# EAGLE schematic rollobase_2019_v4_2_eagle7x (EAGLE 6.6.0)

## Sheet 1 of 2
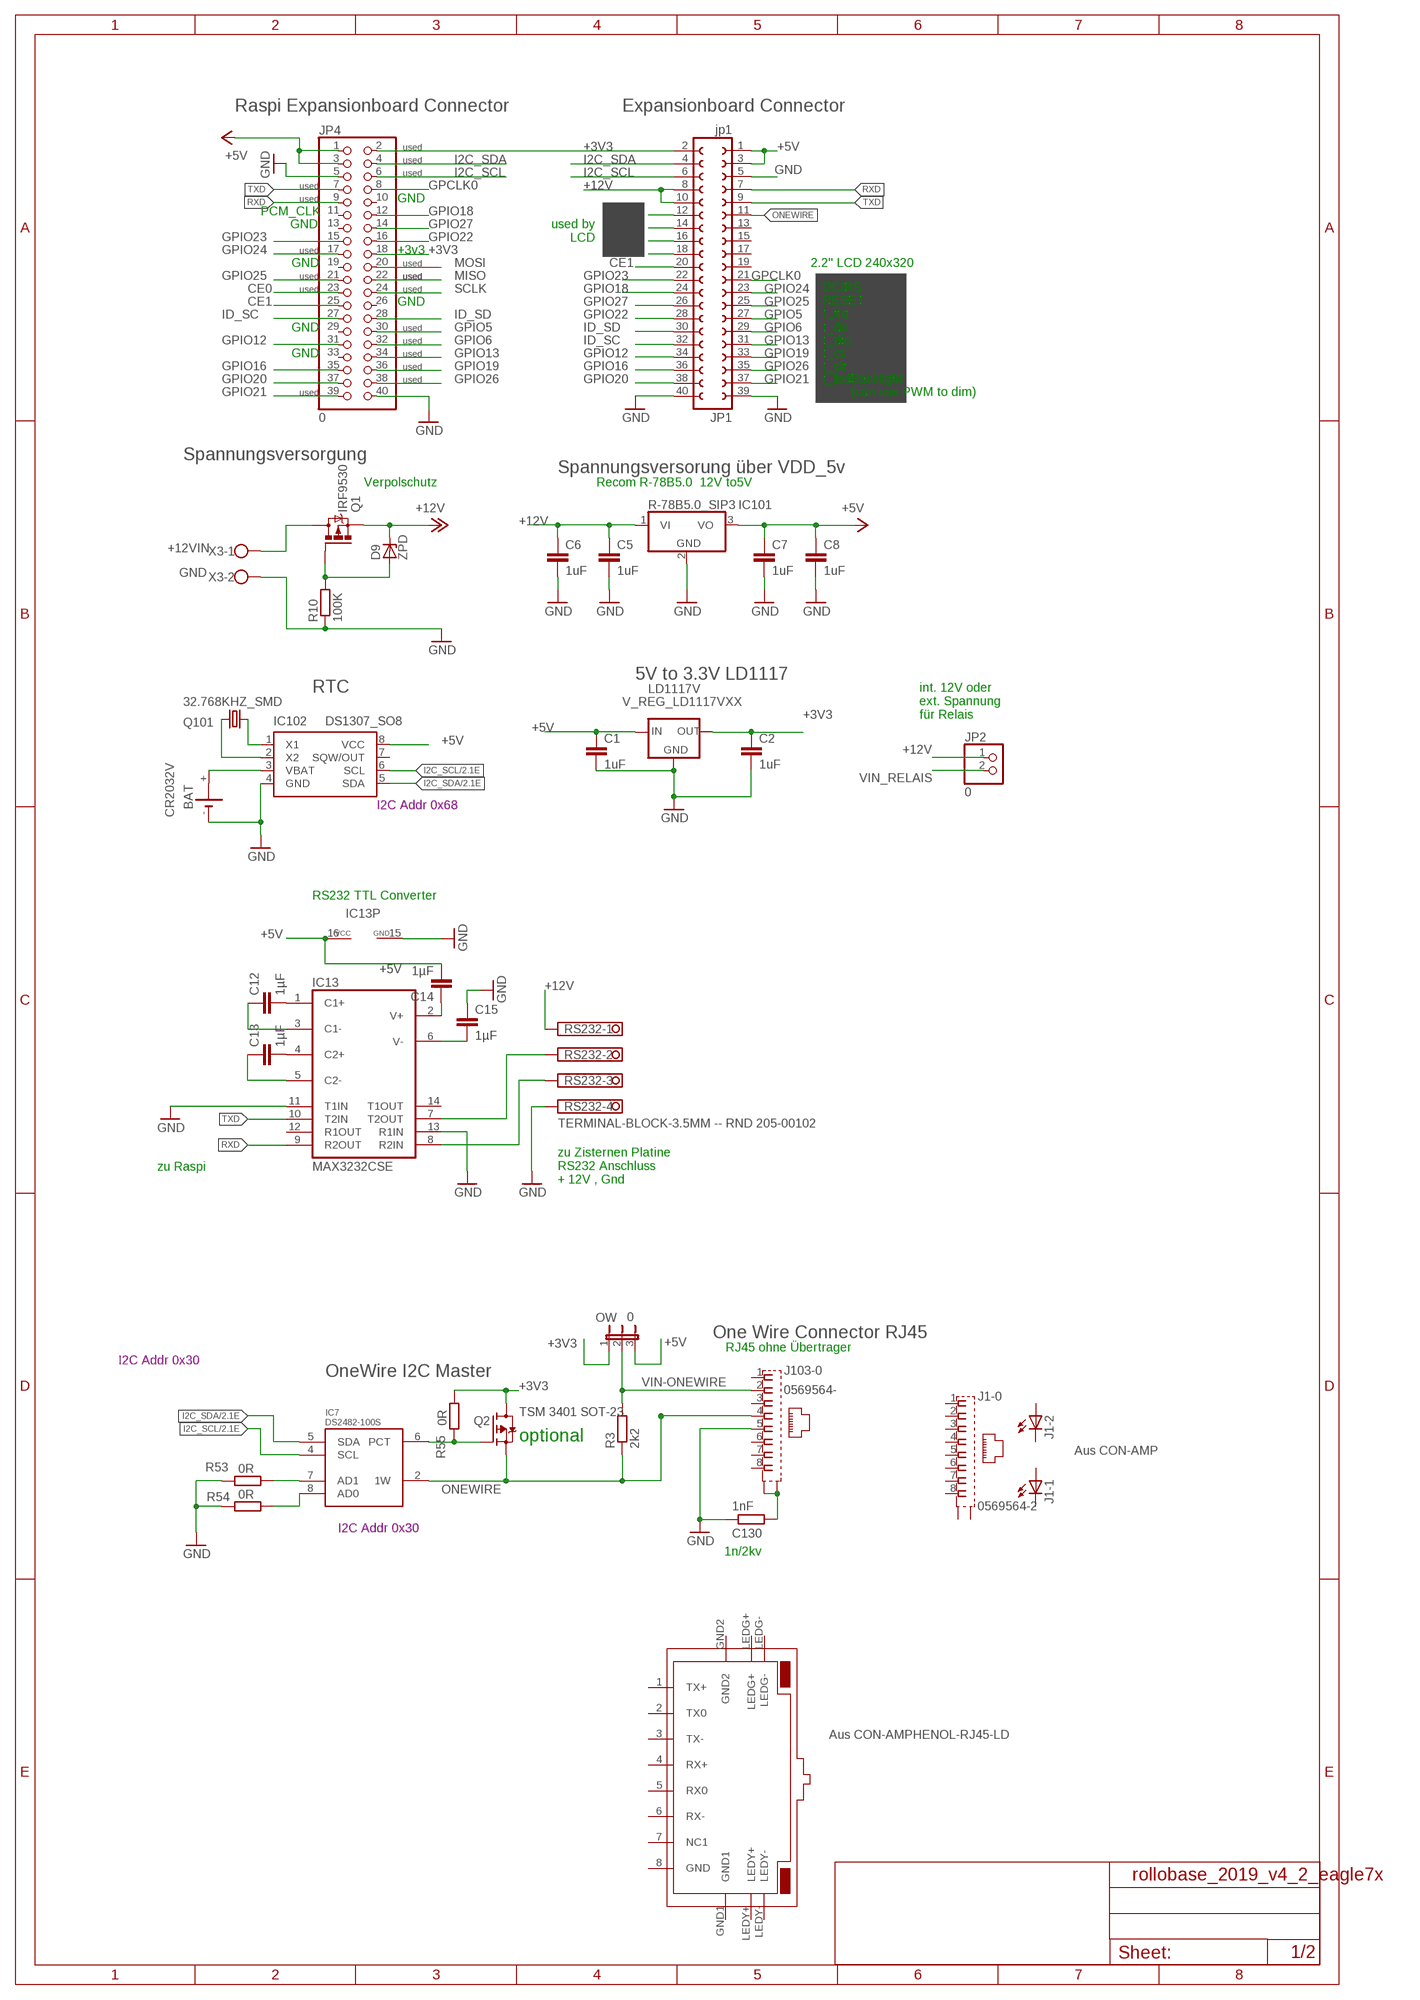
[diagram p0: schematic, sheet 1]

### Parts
BAT  CR2032V  [CR2032V]
C1  1uF  C-EUC1206  [C1206]
C2  1uF  C-EUC1206  [C1206]
C5  1uF  C-EUC1206  [C1206]
C6  1uF  C-EUC1206  [C1206]
C7  1uF  C-EUC1206  [C1206]
C8  1uF  C-EUC1206  [C1206]
C12  1µF  C-EUC1206  [C1206]
C13  1µF  C-EUC1206  [C1206]
C14  1µF  C-EUC1206  [C1206]
C15  1µF  C-EUC1206  [C1206]
C130  1nF  R-EU_R0805  [R0805]
D9  ZPD  [DO35Z10]
IC7  DS2482-100S  [SO08]
IC13  MAX3232CSE  [SO16]
IC101  R-78B5.0_SIP3  [SIP3]
IC102  DS1307_SO8  [SO08]
J1  0569564-2  [0569564]
J103  0569564-  [0569564]
JP1  jp1  FE20-2  [FE20-2]
JP2  0  PINHD-1X2  [1X02]
JP4  0  PINHD-2X20  [2X20]
LD1117V  V_REG_LD1117VXX  [78XXL]
OW  0  JP2E  [JP2]
Q1  IRF9530  [TO220BV]
Q2  TSM 3401 SOT-23  MOSFET-P-SOT23  [SOT23]
Q101  32.768KHZ_SMD  [QSMD]
R3  2k2  R-EU_M1206  [M1206]
R10  100K  R-EU_R1206  [R1206]
R53  0R  R-EU_R1206  [R1206]
R54  0R  R-EU_R1206  [R1206]
R55  0R  R-EU_R1206  [R1206]
RS232  TERMINAL-BLOCK-3.5MM -- RND 205-00102  TERMINAL-BLOCK-3.5MM-4-PIN-ROUND-PAD  [TERMINAL-BLOCK-4-PIN-3.5MM-ROUND-PAD]
U$3  RJ45-TRAFO-L  [RJ45-TRAFO-L]
X3  VERSORGUNG  W237-102  [W237-102]

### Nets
$N5555: C130.1 J103.S1(-0:S1) J103.S2(-0:S2)
+3V3: C2.1 JP1.2 JP4.2 JP4.18 LD1117V.GND(OUT) OW.1 Q2.3(D) R55.1 ; also sheet 2
+5V: C1.1 C7.1 C8.1 C14.2 IC13.16(VCC) IC101.3(VO) IC102.8(VCC) JP1.1 JP1.3 JP4.1 JP4.3 LD1117V.OUT(IN) OW.3
+12V: C5.1 C6.1 D9.C IC101.1(VI) JP1.8 JP1.10 JP2.1 Q1.S RS232.1
+12VIN: Q1.D X3.1
CE0: JP1.18 JP4.23
CE1: JP1.20 JP4.25
GND: BAT.- C1.2 C2.2 C5.2 C6.2 C7.2 C8.2 C15.1 C130.2 IC13.11(T1IN) IC13.13(R1IN) IC13.15(GND) IC101.2(GND) IC102.4(GND) J103.5 JP1.5 JP1.39 JP1.40 JP4.5 JP4.40 LD1117V.IN(GND) R10.1 R53.2 R54.2 RS232.4 X3.2 ; also sheet 2
GPCLK0: JP1.21 JP4.8
GPIO5: JP1.27 JP4.30
GPIO6: JP1.29 JP4.32
GPIO12: JP1.34 JP4.31
GPIO13: JP1.31 JP4.34
GPIO16: JP1.36 JP4.35
GPIO18: JP1.24 JP4.12
GPIO19: JP1.33 JP4.36
GPIO20: JP1.38 JP4.37
GPIO21: JP1.37 JP4.39
GPIO22: JP1.28 JP4.16
GPIO23: JP1.22 JP4.15
GPIO24: JP1.23 JP4.17
GPIO25: JP1.25 JP4.21
GPIO26: JP1.35 JP4.38
GPIO27: JP1.26 JP4.14
I2C_SCL: IC7.4(SCL) IC102.6(SCL) JP1.6 JP4.6 ; also sheet 2
I2C_SDA: IC7.5(SDA) IC102.5(SDA) JP1.4 JP4.4 ; also sheet 2
ID_SC: JP1.32 JP4.27
ID_SD: JP1.30 JP4.28
MISO: JP1.14 JP4.22
MOSI: JP1.12 JP4.20
N$1: IC7.7(AD1) R53.1
N$2: IC7.8(AD0) R54.1
N$12: BAT.+ IC102.3(VBAT)
N$27: IC102.2(X2) Q101.1
N$29: IC102.1(X1) Q101.2
N$35: C12.2 IC13.1(C1+)
N$36: C13.2 IC13.4(C2+)
N$39: C14.1 IC13.2(V+)
N$43: C15.2 IC13.6(V-)
N$44: D9.A Q1.G R10.2
N$52: C12.1 IC13.3(C1-)
N$54: C13.1 IC13.5(C2-)
ONEWIRE: IC7.2(1W) J103.4 JP1.11 Q2.2(S) R3.1
PCTLZ: IC7.6(PCT) Q2.1(G) R55.2
RX: IC13.8(R2IN) RS232.3
RXD: IC13.9(R2OUT) JP1.7 JP4.9
SCLK: JP1.16 JP4.24
TX: IC13.7(T2OUT) RS232.2
TXD: IC13.10(T2IN) JP1.9 JP4.7
VIN-ONEWIRE: J103.2 OW.2 R3.2
VIN_RELAIS: JP2.2 ; also sheet 2
Unconnected: BAT.+@1(+) IC13.12(R1OUT) IC13.14(T1OUT) IC102.7(SQW/OUT) J1.1 J1.2 J1.3 J1.4 J1.5 J1.6 J1.7 J1.8 J1.A1(-1:A) J1.A2(-2:A) J1.C1(-1:C) J1.C2(-2:C) J1.S1(-0:S1) J1.S2(-0:S2) J103.1 J103.3 J103.6 J103.7 J103.8 J103.A1(-1:A) J103.A2(-2:A) J103.C1(-1:C) J103.C2(-2:C) JP1.13 JP1.15 JP1.17 JP1.19 JP4.10 JP4.11 JP4.13 JP4.19 JP4.26 JP4.29 JP4.33 U$3.1(TX+) U$3.2(TX0) U$3.3(TX-) U$3.4(RX+) U$3.5(RX0) U$3.6(RX-) U$3.7(NC1) U$3.LEDG+ U$3.LEDG- U$3.LEDY+ U$3.LEDY-

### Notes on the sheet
- Raspi Expansionboard Connector | Expansionboard Connector
- used
- used
- used
- used
- used | GND
- PCM_CLK
- used by
       LCD
- GND
- used | +3v3
- GND | used | 2.2'' LCD 240x320
- used | used | used
- used | used | DC/RS
- GND | RESET
- t_irq
- GND | used | t_do
- used | t_dio
- GND | used | t_cs
- used | t_clr
- used | t_led
- used
- Backlight
  (can use PWM to dim)
- Spannungsversorgung
- Spannungsversorung über VDD_5v
- Verpolschutz | Recom R-78B5.0 | 12V to5V
- 5V to 3.3V LD1117
- RTC
- int. 12V oder
  ext. Spannung 
  für Relais
- I2C Addr 0x68
- RS232 TTL Converter
- zu Raspi
- zu Zisternen Platine
  RS232 Anschluss
  + 12V , Gnd
- One Wire Connector RJ45
- RJ45 ohne Übertrager
- I2C Addr 0x30
- OneWire I2C Master
- optional
- Aus CON-AMP
- I2C Addr 0x30
- 1n/2kv
- Aus CON-AMPHENOL-RJ45-LD

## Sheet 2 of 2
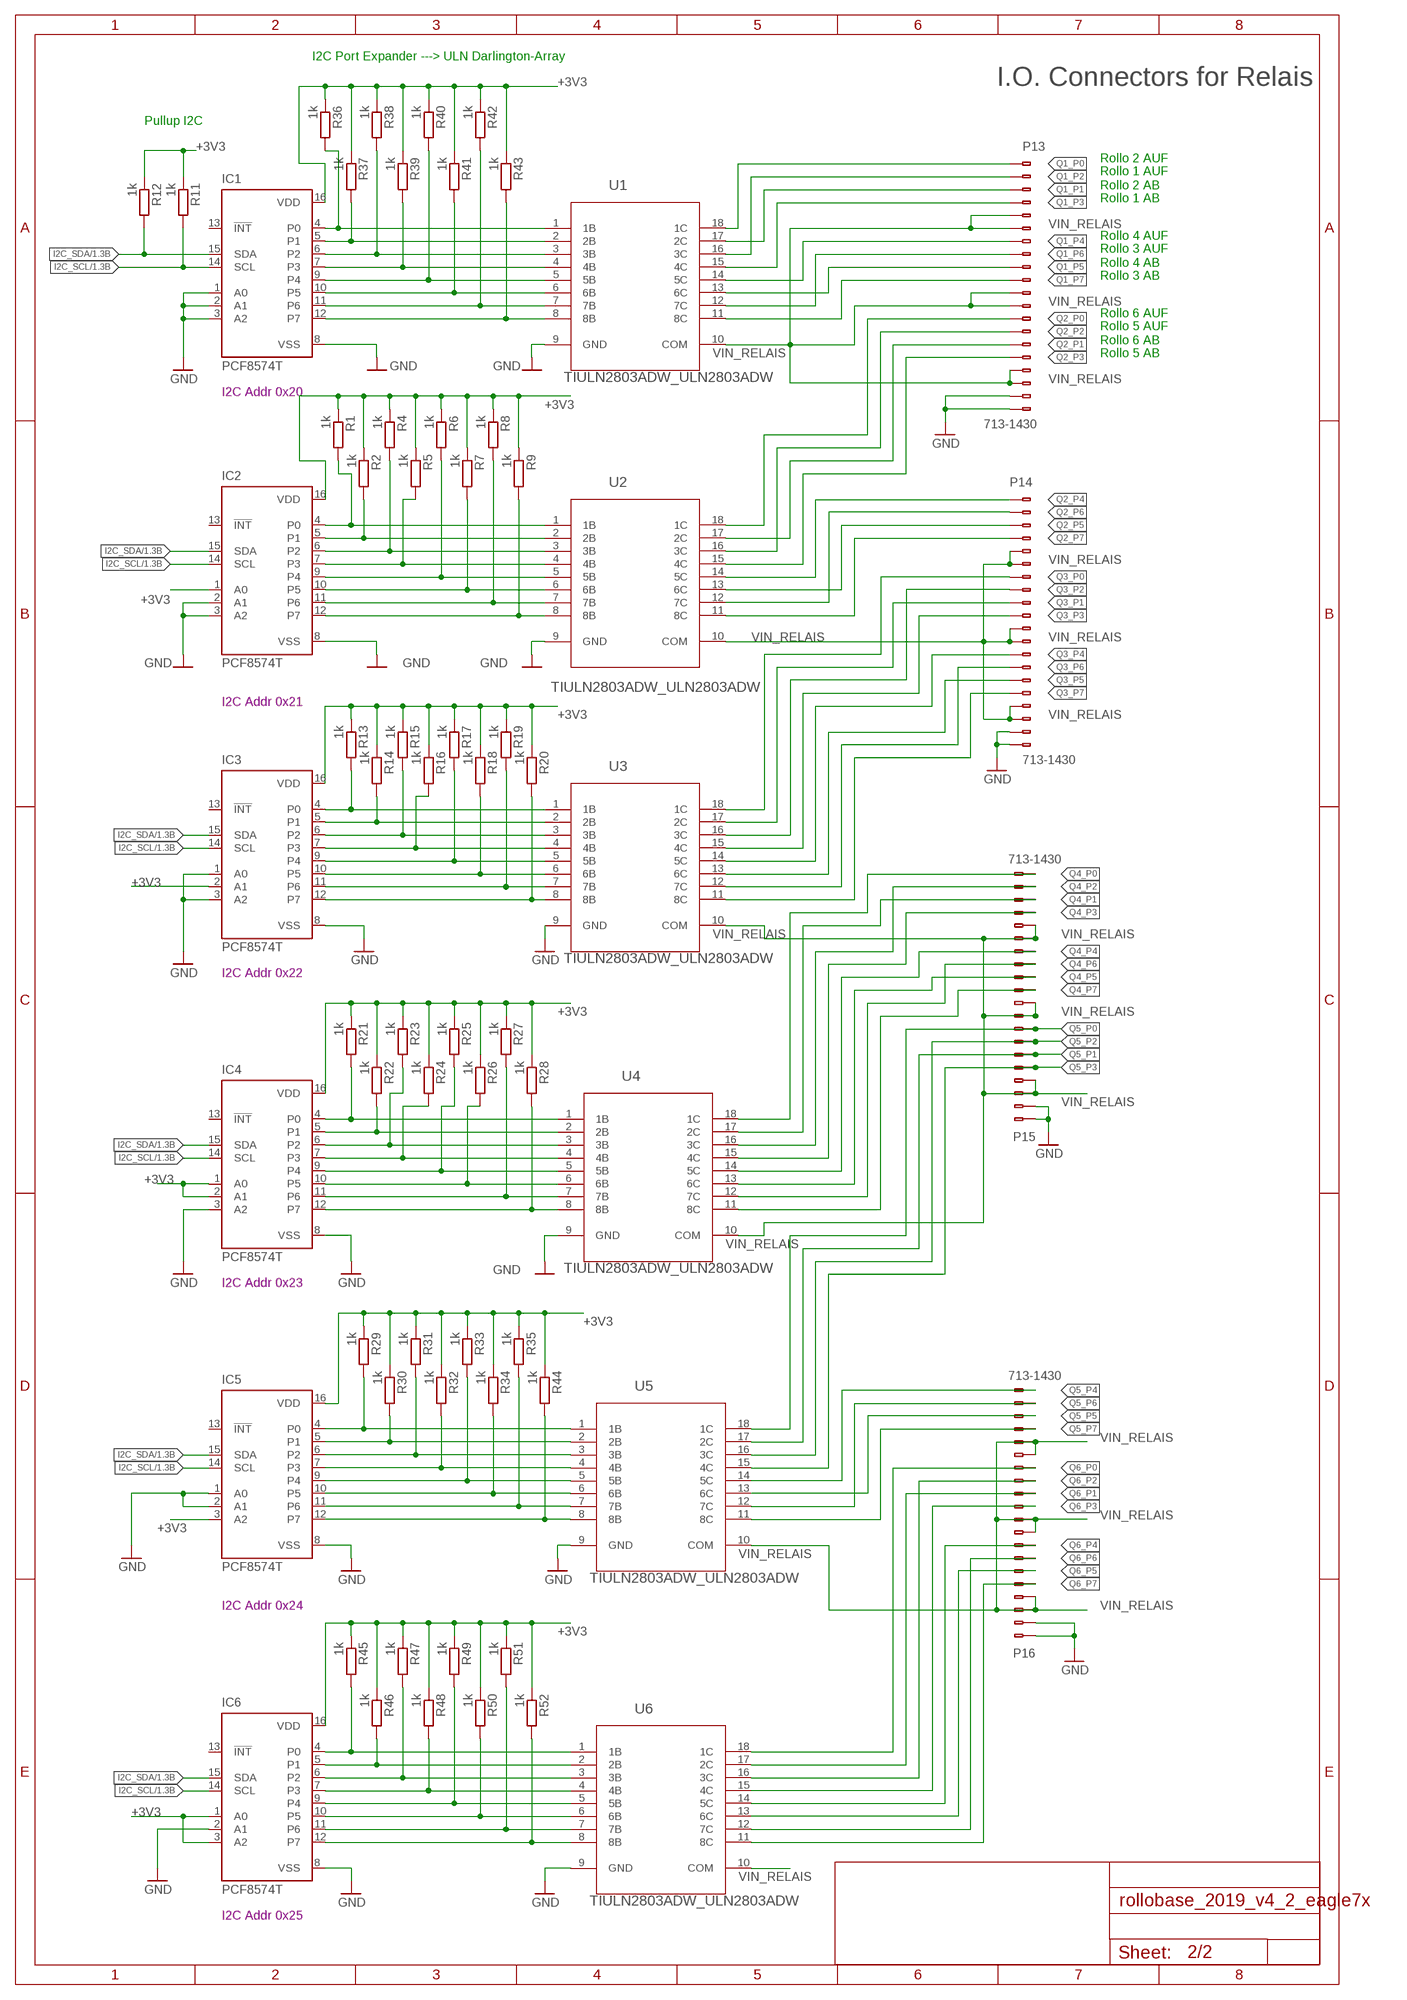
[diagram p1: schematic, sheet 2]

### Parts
IC1  PCF8574T  [SO16W]
IC2  PCF8574T  [SO16W]
IC3  PCF8574T  [SO16W]
IC4  PCF8574T  [SO16W]
IC5  PCF8574T  [SO16W]
IC6  PCF8574T  [SO16W]
P13  713-1430  [713-1425]
P14  713-1430  [713-1425]
P15  713-1430  [713-1425]
P16  713-1430  [713-1425]
R1  1k  R-EU_R0805  [R0805]
R2  1k  R-EU_R0805  [R0805]
R4  1k  R-EU_R0805  [R0805]
R5  1k  R-EU_R0805  [R0805]
R6  1k  R-EU_R0805  [R0805]
R7  1k  R-EU_R0805  [R0805]
R8  1k  R-EU_R0805  [R0805]
R9  1k  R-EU_R0805  [R0805]
R11  1k  R-EU_R1206  [R1206]
R12  1k  R-EU_R1206  [R1206]
R13  1k  R-EU_R0805  [R0805]
R14  1k  R-EU_R0805  [R0805]
R15  1k  R-EU_R0805  [R0805]
R16  1k  R-EU_R0805  [R0805]
R17  1k  R-EU_R0805  [R0805]
R18  1k  R-EU_R0805  [R0805]
R19  1k  R-EU_R0805  [R0805]
R20  1k  R-EU_R0805  [R0805]
R21  1k  R-EU_R0805  [R0805]
R22  1k  R-EU_R0805  [R0805]
R23  1k  R-EU_R0805  [R0805]
R24  1k  R-EU_R0805  [R0805]
R25  1k  R-EU_R0805  [R0805]
R26  1k  R-EU_R0805  [R0805]
R27  1k  R-EU_R0805  [R0805]
R28  1k  R-EU_R0805  [R0805]
R29  1k  R-EU_R0805  [R0805]
R30  1k  R-EU_R0805  [R0805]
R31  1k  R-EU_R0805  [R0805]
R32  1k  R-EU_R0805  [R0805]
R33  1k  R-EU_R0805  [R0805]
R34  1k  R-EU_R0805  [R0805]
R35  1k  R-EU_R0805  [R0805]
R36  1k  R-EU_R0805  [R0805]
R37  1k  R-EU_R0805  [R0805]
R38  1k  R-EU_R0805  [R0805]
R39  1k  R-EU_R0805  [R0805]
R40  1k  R-EU_R0805  [R0805]
R41  1k  R-EU_R0805  [R0805]
R42  1k  R-EU_R0805  [R0805]
R43  1k  R-EU_R0805  [R0805]
R44  1k  R-EU_R0805  [R0805]
R45  1k  R-EU_R0805  [R0805]
R46  1k  R-EU_R0805  [R0805]
R47  1k  R-EU_R0805  [R0805]
R48  1k  R-EU_R0805  [R0805]
R49  1k  R-EU_R0805  [R0805]
R50  1k  R-EU_R0805  [R0805]
R51  1k  R-EU_R0805  [R0805]
R52  1k  R-EU_R0805  [R0805]
U1  TIULN2803ADW_ULN2803ADW  [TIULN2803ADW_SOIC127P1030X265-18N]
U2  TIULN2803ADW_ULN2803ADW  [TIULN2803ADW_SOIC127P1030X265-18N]
U3  TIULN2803ADW_ULN2803ADW  [TIULN2803ADW_SOIC127P1030X265-18N]
U4  TIULN2803ADW_ULN2803ADW  [TIULN2803ADW_SOIC127P1030X265-18N]
U5  TIULN2803ADW_ULN2803ADW  [TIULN2803ADW_SOIC127P1030X265-18N]
U6  TIULN2803ADW_ULN2803ADW  [TIULN2803ADW_SOIC127P1030X265-18N]

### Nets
+3V3: IC1.16(VDD) IC2.1(A0) IC2.16(VDD) IC3.2(A1) IC3.16(VDD) IC4.1(A0) IC4.2(A1) IC4.16(VDD) IC5.3(A2) IC5.16(VDD) IC6.1(A0) IC6.3(A2) IC6.16(VDD) R1.1 R2.1 R4.1 R5.1 R6.1 R7.1 R8.1 R9.1 R11.1 R12.1 R13.1 R14.1 R15.1 R16.1 R17.1 R18.1 R19.1 R20.1 R21.1 R22.1 R23.1 R24.1 R25.1 R26.1 R27.1 R28.1 R29.1 R30.1 R31.1 R32.1 R33.1 R34.1 R35.1 R36.1 R37.1 R38.1 R39.1 R40.1 R41.1 R42.1 R43.1 R44.1 R45.1 R46.1 R47.1 R48.1 R49.1 R50.1 R51.1 R52.1 ; also sheet 1
GND: IC1.1(A0) IC1.2(A1) IC1.3(A2) IC1.8(VSS) IC2.2(A1) IC2.3(A2) IC2.8(VSS) IC3.1(A0) IC3.3(A2) IC3.8(VSS) IC4.3(A2) IC4.8(VSS) IC5.1(A0) IC5.2(A1) IC5.8(VSS) IC6.2(A1) IC6.8(VSS) P13.19(B-19) P13.20(B-20) P14.19(B-19) P14.20(B-20) P15.1(B-1) P15.2(B-2) P16.1(B-1) P16.2(B-2) U1.9(GND) U2.9(GND) U3.9(GND) U4.9(GND) U5.9(GND) U6.9(GND) ; also sheet 1
I2C_SCL: IC1.14(SCL) IC2.14(SCL) IC3.14(SCL) IC4.14(SCL) IC5.14(SCL) IC6.14(SCL) R11.2 ; also sheet 1
I2C_SDA: IC1.15(SDA) IC2.15(SDA) IC3.15(SDA) IC4.15(SDA) IC5.15(SDA) IC6.15(SDA) R12.2 ; also sheet 1
IC1_P1: IC1.5(P1) R37.2 U1.2(2B)
IC1_P2: IC2.5(P1) R2.2 U2.2(2B)
IC1_P3: IC2.4(P0) R1.2 U2.1(1B)
IC1_P4: IC2.6(P2) R4.2 U2.3(3B)
IC1_P5: IC2.7(P3) R5.2 U2.4(4B)
IC1_P6: IC2.9(P4) R6.2 U2.5(5B)
IC1_P7: IC2.10(P5) R7.2 U2.6(6B)
IC1_P8: IC2.11(P6) R8.2 U2.7(7B)
IC1_P9: IC1.4(P0) R36.2 U1.1(1B)
IC1_P10: IC1.6(P2) R38.2 U1.3(3B)
IC1_P11: IC1.7(P3) R39.2 U1.4(4B)
IC1_P12: IC1.9(P4) R40.2 U1.5(5B)
IC1_P13: IC1.10(P5) R41.2 U1.6(6B)
IC1_P14: IC1.11(P6) R42.2 U1.7(7B)
IC1_P15: IC1.12(P7) R43.2 U1.8(8B)
IC1_P16: IC2.12(P7) R9.2 U2.8(8B)
IC1_P17: IC3.5(P1) R14.2 U3.2(2B)
IC1_P18: IC3.4(P0) R13.2 U3.1(1B)
IC1_P19: IC3.6(P2) R15.2 U3.3(3B)
IC1_P20: IC3.7(P3) R16.2 U3.4(4B)
IC1_P21: IC3.9(P4) R17.2 U3.5(5B)
IC1_P22: IC3.10(P5) R18.2 U3.6(6B)
IC1_P23: IC3.11(P6) R19.2 U3.7(7B)
IC1_P24: IC3.12(P7) R20.2 U3.8(8B)
IC1_P25: IC4.5(P1) R22.2 U4.2(2B)
IC1_P26: IC4.4(P0) R21.2 U4.1(1B)
IC1_P27: IC4.6(P2) R23.2 U4.3(3B)
IC1_P28: IC4.7(P3) R24.2 U4.4(4B)
IC1_P29: IC4.9(P4) R25.2 U4.5(5B)
IC1_P30: IC4.10(P5) R26.2 U4.6(6B)
IC1_P31: IC4.11(P6) R27.2 U4.7(7B)
IC1_P32: IC4.12(P7) R28.2 U4.8(8B)
IC1_P33: IC5.5(P1) R30.2 U5.2(2B)
IC1_P34: IC5.4(P0) R29.2 U5.1(1B)
IC1_P35: IC5.6(P2) R31.2 U5.3(3B)
IC1_P36: IC5.7(P3) R32.2 U5.4(4B)
IC1_P37: IC5.9(P4) R33.2 U5.5(5B)
IC1_P38: IC5.10(P5) R34.2 U5.6(6B)
IC1_P39: IC5.11(P6) R35.2 U5.7(7B)
IC1_P40: IC5.12(P7) R44.2 U5.8(8B)
IC6_P0: IC6.4(P0) R45.2 U6.1(1B)
IC6_P1: IC6.5(P1) R46.2 U6.2(2B)
IC6_P2: IC6.6(P2) R47.2 U6.3(3B)
IC6_P3: IC6.7(P3) R48.2 U6.4(4B)
IC6_P4: IC6.9(P4) R49.2 U6.5(5B)
IC6_P5: IC6.10(P5) R50.2 U6.6(6B)
IC6_P6: IC6.11(P6) R51.2 U6.7(7B)
IC6_P7: IC6.12(P7) R52.2 U6.8(8B)
Q1_P0: P13.1(B-1) U1.18(1C)
Q1_P1: P13.3(B-3) U1.17(2C)
Q1_P2: P13.2(B-2) U1.16(3C)
Q1_P3: P13.4(B-4) U1.15(4C)
Q1_P4: P13.7(B-7) U1.14(5C)
Q1_P5: P13.9(B-9) U1.13(6C)
Q1_P6: P13.8(B-8) U1.12(7C)
Q1_P7: P13.10(B-10) U1.11(8C)
Q2_P0: P13.13(B-13) U2.18(1C)
Q2_P1: P13.15(B-15) U2.17(2C)
Q2_P2: P13.14(B-14) U2.16(3C)
Q2_P3: P13.16(B-16) U2.15(4C)
Q2_P4: P14.1(B-1) U2.14(5C)
Q2_P5: P14.3(B-3) U2.13(6C)
Q2_P6: P14.2(B-2) U2.12(7C)
Q2_P7: P14.4(B-4) U2.11(8C)
Q3_P0: P14.7(B-7) U3.18(1C)
Q3_P1: P14.9(B-9) U3.17(2C)
Q3_P2: P14.8(B-8) U3.16(3C)
Q3_P3: P14.10(B-10) U3.15(4C)
Q3_P4: P14.13(B-13) U3.14(5C)
Q3_P5: P14.15(B-15) U3.13(6C)
Q3_P6: P14.14(B-14) U3.12(7C)
Q3_P7: P14.16(B-16) U3.11(8C)
Q4_P0: P15.20(B-20) U4.18(1C)
Q4_P1: P15.18(B-18) U4.17(2C)
Q4_P2: P15.19(B-19) U4.16(3C)
Q4_P3: P15.17(B-17) U4.15(4C)
Q4_P4: P15.14(B-14) U4.14(5C)
Q4_P5: P15.12(B-12) U4.13(6C)
Q4_P6: P15.13(B-13) U4.12(7C)
Q4_P7: P15.11(B-11) U4.11(8C)
Q5_P0: P15.8(B-8) U5.18(1C)
Q5_P1: P15.6(B-6) U5.17(2C)
Q5_P2: P15.7(B-7) U5.16(3C)
Q5_P3: P15.5(B-5) U5.15(4C)
Q5_P4: P16.20(B-20) U5.14(5C)
Q5_P5: P16.18(B-18) U5.13(6C)
Q5_P6: P16.19(B-19) U5.12(7C)
Q5_P7: P16.17(B-17) U5.11(8C)
Q6_P0: P16.14(B-14) U6.18(1C)
Q6_P1: P16.12(B-12) U6.17(2C)
Q6_P2: P16.13(B-13) U6.16(3C)
Q6_P3: P16.11(B-11) U6.15(4C)
Q6_P4: P16.8(B-8) U6.14(5C)
Q6_P5: P16.6(B-6) U6.13(6C)
Q6_P6: P16.7(B-7) U6.12(7C)
Q6_P7: P16.5(B-5) U6.11(8C)
VIN_RELAIS: P13.5(B-5) P13.6(B-6) P13.11(B-11) P13.12(B-12) P13.17(B-17) P13.18(B-18) P14.5(B-5) P14.6(B-6) P14.11(B-11) P14.12(B-12) P14.17(B-17) P14.18(B-18) P15.3(B-3) P15.4(B-4) P15.9(B-9) P15.10(B-10) P15.15(B-15) P15.16(B-16) P16.3(B-3) P16.4(B-4) P16.9(B-9) P16.10(B-10) P16.15(B-15) P16.16(B-16) U1.10(COM) U2.10(COM) U3.10(COM) U4.10(COM) U5.10(COM) U6.10(COM) ; also sheet 1
Unconnected: IC1.13(!INT) IC2.13(!INT) IC3.13(!INT) IC4.13(!INT) IC5.13(!INT) IC6.13(!INT)

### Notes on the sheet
- I2C Port Expander ---> ULN Darlington-Array
- I.O. Connectors for Relais
- Pullup I2C
- Rollo 2 AUF
  
  Rollo 2 AB
- Rollo 1 AUF
  
  Rollo 1 AB
- Rollo 4 AUF
  
  Rollo 4 AB
- Rollo 3 AUF
  
  Rollo 3 AB
- Rollo 6 AUF
  
  Rollo 6 AB
- Rollo 5 AUF
  
  Rollo 5 AB
- I2C Addr 0x20
- I2C Addr 0x21
- I2C Addr 0x22
- I2C Addr 0x23
- I2C Addr 0x24
- I2C Addr 0x25

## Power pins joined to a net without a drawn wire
GND: IC7.3(GND) U$3.8(GND)
GND1: U$3.GND1
GND2: U$3.GND2
VDD: IC7.1(VDD)

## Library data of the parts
BAT = battery:CR2032V: LI BATTERY Varta
C1 C2 C5-C8 = resistor:C-EU: CAPACITOR, European symbol
C12-C15 = rcl:C-EU: CAPACITOR, European symbol
C130 R10-R12 R53-R55 = resistor:R-EU_: RESISTOR, European symbol
D9 = diode:ZPD: Z DIODE
IC1-IC6 = micro-philips:PCF8574: I2C-Bus Remote 8-bit I/O expander http://www.semiconductors.philips.com/acrobat_download/datasheets/PCF8574_4.pdf; MPN: PCF8574T/3,512; OC_FARNELL: 1201255; OC_NEWARK: 70R6870
IC7 = 1wire:DS2482-100: I2C to 1-Wire Host Adapter/Line Driver This device is a onewire host and I2C interface in one chip. It provides the complete DC/AC requirements for onewire communication, including overdrive speed mode, but, unlike the DS2480B chip, no 12V EPROM programming. Notes: For overdrive speed and 5V EEPROM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
IC13 = maxim:MAX3232*: True RS-232 Transceivers 3.0V to 5.5V, Low-Power up to 1Mbps, Using Four 0.1µF External Capacitors Source: http://pdfserv.maxim-ic.com/en/ds/MAX3222-MAX3241.pdf
IC101 = dc-dc-schaltregler:R-78B5.0_SIP3: 204953
IC102 = maxim:DS1307_SO8: 207082
J1 = con-amp:0569564-*: MODULAR JACK 8 POS., RIGHT ANGLE, LOW PROFILE WITH LEDS Source: http://ecommas.tycoelectronics.com/.. 569564_K.pdf
J103 = con_rj45:0569564-*: 204948
JP1 = con-lsta:FE20-2: FEMALE HEADER; OC_FARNELL: unknown; OC_NEWARK: unknown
JP2 = pinhead:PINHD-1X2: PIN HEADER
JP4 = pinhead:PINHD-2X20: PIN HEADER
LD1117V = SparkFun-PowerIC:V_REG_LD1117VXX: LD1117VXX voltage regulator. We carry the 3.3V version (COM-00526) in TO-220 package.
OW = jumper:JP2E: JUMPER
P13-P16 = con-wago255:713-1430
Q1 = transistor-power:IRF9530: P-CHANNEL HEXFET POWER-MOS-FET Source: http://www.irf.com/product-info/datasheets/data/irf9530.pdf
Q2 = we-transistor:MOSFET-P: P-Channel MOSFET SOT23 P-Chn MOSFET TSM3401, IRLML6402 (Vds>=20V, Id>=2A + Rds<=0.1Ohm @ Vgs=4.5V)
Q101 = quarz:32.768KHZ_SMD: 207083
R1-R9 R13-R52 = rcl:R-EU_: RESISTOR, European symbol
RS232 = Rembrandt Electronics - Terminal Block 3-5mm v1-0:TERMINAL-BLOCK-3.5MM-4-PIN: Terminal Block 3.5mm Pitch: 3,5 mm Number of pins: 4 Created by Rembrandt Electronics www.rembrandtelectronics.com
U1-U6 = uln2803-test:TIULN2803ADW_ULN2803ADW: Darlington transistor array; MPN: ULN2803ADW; OC_FARNELL: 1652419; OC_NEWARK: 69K0711; PACKAGE: SOIC-18; SUPPLIER: TEXAS INSTRUMENTS
U$3 = con-amphenol-rj45-ld:RJ45-TRAFO-L: RJ45 socket with integrated magnetics and LEDs Naming: AmphenolLMJ1998824110DL1T39J TMERJ45-TRAFO-L Author: Petr Kalandra Datasheet: http://zefiryn.tme.pl/dok/zlacza/rjtrafol.PDF
X3 = con-wago-500:W237-102: WAGO SCREW CLAMP; MPN: 237-102; OC_FARNELL: unknown; OC_NEWARK: 70K9898

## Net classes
0 default: clearance 0.203 mm
1 signal: width 0.406 mm, drill 0.254 mm, clearance 0.203 mm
